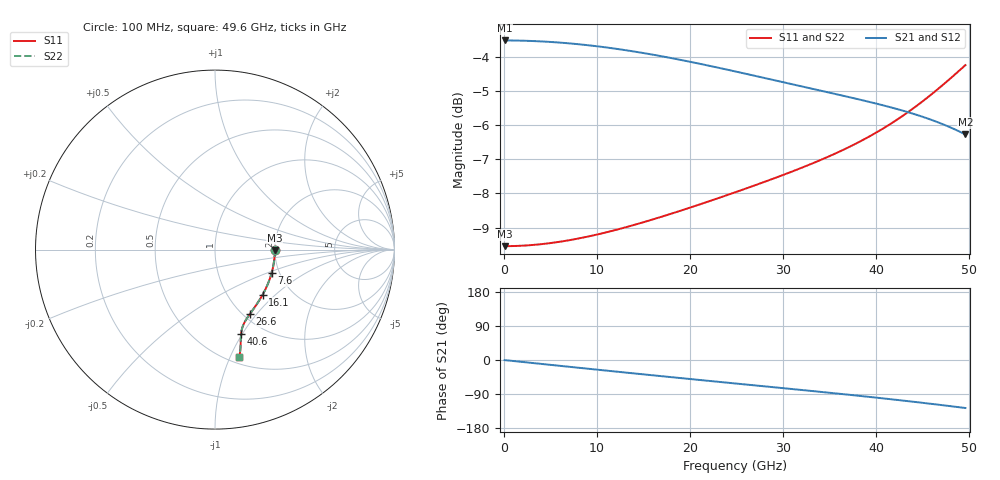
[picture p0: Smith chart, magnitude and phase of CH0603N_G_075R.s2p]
# GHz S RI R 75
! S-Parameters data
! Freq  reS11  imS11  reS21  imS21  reS12  imS12  reS22  imS22
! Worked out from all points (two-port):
!   100 points, 100 MHz to 49.6 GHz, reference 75 ohm
!   highest |S21| = -3.52 dB at 100 MHz (marker M1); lowest = -6.3 dB at 49.6 GHz (marker M2)
!   |S21| within 3 dB of the highest: start of sweep to end of sweep
!   lowest |S11| = -9.5 dB at 100 MHz (marker M3), VSWR 2.00, Z = 150 - j0.589 ohm
!   |S11| at or under -10 dB: nowhere
!   |S22| runs from -9.5 to -4.2 dB; largest |S21 - S12| = 0
!   S11 on the Smith chart (normalised r, x): 100 MHz: 2.00, -0.01; 7.6 GHz: 1.82, -0.53; 16.1 GHz: 1.44, -0.83; 26.6 GHz: 1.08, -0.92; 40.6 GHz: 0.79, -0.99; 49.6 GHz: 0.56, -1.08
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0.1  0.3333 -0.00175  0.6667 -0.00297  0.6667 -0.00297  0.3333 -0.00175
3.6  0.3293 -0.0624  0.6564 -0.106  0.6564 -0.106  0.3293 -0.0624
5.6  0.3237 -0.0962  0.6421 -0.1632  0.6421 -0.1632  0.3237 -0.0962
7.6  0.3159 -0.1289  0.622 -0.2181  0.622 -0.2181  0.3159 -0.1289
8.6  0.3113 -0.1448  0.6098 -0.2445  0.6098 -0.2445  0.3113 -0.1448
12.1  0.292 -0.1971  0.5577 -0.3303  0.5577 -0.3303  0.292 -0.1971
16.1  0.2659 -0.2502  0.4825 -0.4131  0.4825 -0.4131  0.2659 -0.2502
16.6  0.2624 -0.2563  0.4722 -0.4222  0.4722 -0.4222  0.2624 -0.2563
18.6  0.2485 -0.2797  0.4293 -0.4556  0.4293 -0.4556  0.2485 -0.2797
20.6  0.2345 -0.3014  0.3841 -0.4843  0.3841 -0.4843  0.2345 -0.3014
22.6  0.2208 -0.3215  0.3373 -0.5083  0.3373 -0.5083  0.2208 -0.3215
25.1  0.2045 -0.3446  0.2773 -0.5317  0.2773 -0.5317  0.2045 -0.3446
26.6  0.1953 -0.3576  0.2407 -0.5424  0.2407 -0.5424  0.1953 -0.3576
29.6  0.1785 -0.382  0.167 -0.5564  0.167 -0.5564  0.1785 -0.382
33.1  0.1627 -0.409  0.0809 -0.5609  0.0809 -0.5609  0.1627 -0.409
37.1  0.1506 -0.4405  -0.0169 -0.5505  -0.0169 -0.5505  0.1506 -0.4405
40.6  0.1454 -0.4722  -0.101 -0.5268  -0.101 -0.5268  0.1454 -0.4722
41.6  0.1446 -0.4825  -0.1246 -0.5173  -0.1246 -0.5173  0.1446 -0.4825
43.6  0.1437 -0.5055  -0.1706 -0.4941  -0.1706 -0.4941  0.1437 -0.5055
45.6  0.1427 -0.5323  -0.2143 -0.4652  -0.2143 -0.4652  0.1427 -0.5323
47.6  0.1404 -0.5632  -0.2547 -0.4303  -0.2547 -0.4303  0.1404 -0.5632
49.6  0.1354 -0.5984  -0.29 -0.3896  -0.29 -0.3896  0.1354 -0.5984
